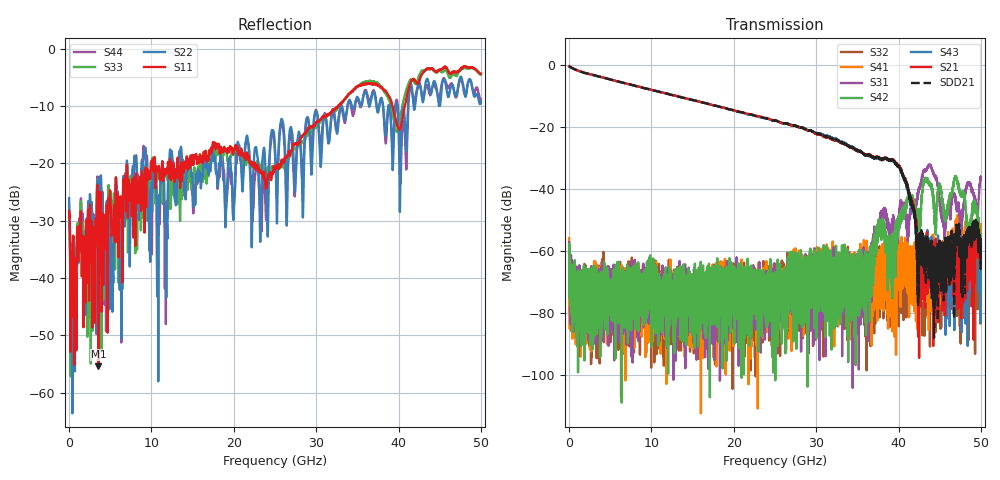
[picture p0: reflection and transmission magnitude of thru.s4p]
!Keysight Technologies,N5245A,MY49151038,A.10.64.09
!Date: Tuesday, August 13, 2019 16:00:19
!Correction: S11(Full 4 Port(1,2,3,4))
!S12(Full 4 Port(1,2,3,4))
!S13(Full 4 Port(1,2,3,4))
!S14(Full 4 Port(1,2,3,4))
!S21(Full 4 Port(1,2,3,4))
!S22(Full 4 Port(1,2,3,4))
!S23(Full 4 Port(1,2,3,4))
!S24(Full 4 Port(1,2,3,4))
!S31(Full 4 Port(1,2,3,4))
!S32(Full 4 Port(1,2,3,4))
!S33(Full 4 Port(1,2,3,4))
!S34(Full 4 Port(1,2,3,4))
!S41(Full 4 Port(1,2,3,4))
!S42(Full 4 Port(1,2,3,4))
!S43(Full 4 Port(1,2,3,4))
!S44(Full 4 Port(1,2,3,4))
!S4P File: Measurements: <S11,S12,S13,S14>,
!<S21,S22,S23,S24>,
!<S31,S32,S33,S34>,
!<S41,S42,S43,S44>:
# Hz S  MA  R 50
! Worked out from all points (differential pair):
!   5000 points, 10 MHz to 50 GHz, reference 50 ohm
!   strongest paths, dB at 10 MHz, 12.51 GHz, 25.01 GHz, 37.51 GHz, 50 GHz:
!     S21: -0.3, -9.6, -17.8, -29.7, -63.9
!     S43: -0.3, -9.6, -17.9, -30.0, -59.0
!     S42: -65.9, -73.4, -80.8, -55.2, -57.3
!     S31: -57.2, -76.3, -71.2, -53.6, -36.1
!     S41: -55.8, -70.3, -68.7, -65.2, -52.7
!     S32: -57.6, -90.1, -72.0, -64.0, -62.3
!   taken as a pair (ports 1,3 in; 2,4 out), SDD21 dB: -0.3, -9.6, -17.9, -29.8, -57.3
!   lowest |S11| = -55.4 dB at 3.56 GHz (marker M1), VSWR 1.00, Z = 50.1 - j0.137 ohm
!   |S11| at or under -10 dB: start of sweep to 32.64 GHz; 39.27 GHz to 40.76 GHz (1.495 GHz wide, 3.73 % of centre)
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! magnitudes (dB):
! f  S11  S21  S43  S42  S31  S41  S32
! 10 MHz  -28.3  -0.3  -0.3  -65.9  -57.2  -55.8  -57.6
! 3.56 GHz  -55.4  -3.5  -3.6  -72.8  -73.2  -79.1  -81.7
! 35.21 GHz  -6.4  -27.8  -27.7  -81.0  -63.0  -81.0  -68.7
! 40.16 GHz  -14.0  -32.8  -33.3  -52.1  -46.5  -61.5  -69.6
! 43.34 GHz  -3.7  -66.8  -56.1  -37.0  -33.9  -66.1  -67.2
! 45.53 GHz  -3.2  -66.1  -64.9  -47.6  -51.4  -59.9  -67.9
! 50 GHz  -4.4  -63.9  -59.0  -57.3  -36.1  -52.7  -62.3
